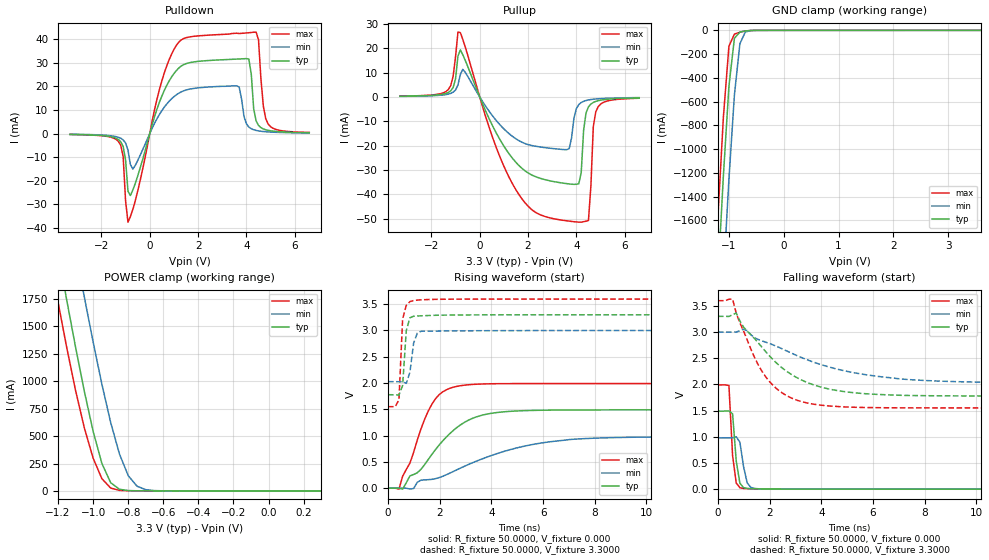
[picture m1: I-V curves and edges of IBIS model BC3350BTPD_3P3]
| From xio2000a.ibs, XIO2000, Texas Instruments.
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|   Model BC3350BTPD_3P3
[Model]   BC3350BTPD_3P3
Model_type   I/O
Polarity   Non-Inverting
Enable   Active-Low
Vinl =   0.9900V
Vinh =   2.3100V
Vmeas =   1.6500V
Cref =  15.0000pF
Rref = 100.0000M
Vref =  0.000V
C_comp   1.9708pF   2.0638pF   1.9731pF
[Model Spec]
|   typ   min   max
Vinh   2.31V   2.10V   2.52V
Vinl   0.99V   0.90V   1.08V
Vmeas   1.65V   1.50V   1.80V
[Temperature Range]   25.0000   0.1250k   -40.0000
[Voltage Range]   3.3000V   3.0000V   3.6000V
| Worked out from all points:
|   slope of the pulldown table from 0 to 0.495 V, typ, clamps not added: 31.4 ohm
|   slope of the pullup table from 0 to 0.495 V, typ, clamps not added: 44.5 ohm
|   GND clamp passes 1 mA (typ) near -0.59 V on its own axis
|   POWER clamp passes 1 mA (typ) near -0.74 V on its own axis
|   rising waveform, R_fixture 50.0000, V_fixture 0.000: 20-80 % time 1.63ns typ, 3.19ns min, 936ps max; typ from 0 V to 1.49 V
|   rising waveform, R_fixture 50.0000, V_fixture 3.3000: 20-80 % time 123ps typ, 174ps min, 113ps max; typ from 1.78 V to 3.3 V
|   falling waveform, R_fixture 50.0000, V_fixture 0.000: 20-80 % time 182ps typ, 214ps min, 166ps max; typ from 1.49 V to 0 V
|   falling waveform, R_fixture 50.0000, V_fixture 3.3000: 20-80 % time 2.06ns typ, 3.41ns min, 1.34ns max; typ from 3.3 V to 1.78 V
[Pulldown]
| voltage   I(typ)   I(min)   I(max)
-3.3V     -363uA     -290uA     -391uA
-1.3V     -2.499mA   -1.558mA   -3.272mA
-1.1V     -5.495mA   -2.672mA   -9.754mA
-900mV    -24.57mA   -7.086mA   -37.63mA
-700mV    -23.98mA   -15.08mA   -32.22mA
400mV     13.29mA    8.099mA    18.71mA
1.1V      26.74mA    16.46mA    37.45mA
3.6V      31.62mA    20.28mA    42.61mA
4.1V      31.65mA    2.775mA    42.82mA
4.4V      5.419mA    1.337mA    43.09mA
4.9V      1.364mA    701uA      4.046mA
6.6V      366uA      264uA      482uA
[Pullup]
| voltage   I(typ)   I(min)   I(max)
-3.3V     276uA      223uA      319uA
-1.3V     1.831mA    1.157mA    3.006mA
-800mV    19.29mA    9.256mA    26.38mA
600mV     -13.2mA    -8.655mA   -18.5mA
1.6V      -27.94mA   -17.82mA   -39.75mA
3.7V      -35.73mA   -21.26mA   -51mA
4.2V      -31.01mA   -2.304mA   -51.44mA
4.3V      -13.58mA   -1.804mA   -51.23mA
4.5V      -4.094mA   -1.249mA   -50.72mA
4.7V      -2.272mA   -950.1uA   -12.21mA
4.9V      -1.556mA   -765.1uA   -4.03mA
6.6V      -413uA     -285uA     -544uA
[GND_clamp]
| voltage   I(typ)   I(min)   I(max)
-3.3V     -22.46A    -23.25A    -22.02A
-1.3V     -2.981A    -3.864A    -2.466A
-1.2V     -2.075A    -2.956A    -1.561A
-1.1V     -1.216A    -2.078A    -723.4mA
-1V       -470.1mA   -1.253A    -133.5mA
-900mV    -66.75mA   -544.3mA   -31.76mA
-800mV    -14.28mA   -112.3mA   -15.85mA
-700mV    -5.191mA   -13.11mA   -5.235mA
-600mV    -1.114mA   -2.329mA   -804.1uA
-400mV    -42.11uA   -65.68uA   -59.17uA
3.6V      0A         0A         0A
[POWER_clamp]
| voltage   I(typ)   I(min)   I(max)
-3.3V     22.56A     23.38A     22.11A
-1.25V    2.627A     3.53A      2.158A
-1.2V     2.177A     3.077A     1.722A
-1.15V    1.736A     2.631A     1.304A
-1.05V    907.7mA    1.767A     573.9mA
-1V       543.7mA    1.358A     298.8mA
-950mV    250.4mA    972.4mA    111.3mA
-900mV    75.01mA    624.5mA    26.23mA
-850mV    15.11mA    336.8mA    5.041mA
-800mV    3.129mA    139.7mA    1.712mA
-750mV    1.084mA    43.46mA    1.075mA
300mV     0A         0A         0A
[Ramp]
| variable   typ   min   max
dV/dt_r   0.8935/1.6105n   0.5876/3.1587n   1.1937/0.9264n
dV/dt_f   0.9123/2.0434n   0.5823/3.3754n   1.2278/1.3245n
R_load = 50.0000
[Rising Waveform]
R_fixture = 50.0000
V_fixture = 0.000
V_fixture_min = 0.000
V_fixture_max = 0.000
| time   V(typ)   V(min)   V(max)
0s        1.533nV    33.95nV    723.3pV
424.2ps   2.21mV     -92.99uV   -18.02mV
565.7ps   -18.48mV   718.1uV    226.7mV
848.5ps   234.3mV    -16.16mV   476.1mV
1.273ns   357.1mV    151.2mV    1.122V
1.697ns   642.6mV    168mV      1.597V
2.546ns   1.106V     322.6mV    1.923V
3.818ns   1.408V     589.6mV    1.984V
6.364ns   1.485V     888.4mV    1.99V
14ns      1.489V     979.4mV    1.99V
[Rising Waveform]
R_fixture = 50.0000
V_fixture = 3.3000
V_fixture_min = 3.0000
V_fixture_max = 3.6000
| time   V(typ)   V(min)   V(max)
0s        1.777V     2.026V     1.55V
282.8ps   1.776V     2.026V     1.55V
424.2ps   1.77V      2.024V     1.684V
565.7ps   1.952V     2.026V     3.216V
707.1ps   2.997V     1.994V     3.477V
848.5ps   3.241V     2.205V     3.548V
989.9ps   3.27V      2.755V     3.568V
1.131ns   3.275V     2.946V     3.577V
1.273ns   3.278V     2.983V     3.582V
14ns      3.298V     2.999V     3.597V
[Falling Waveform]
R_fixture = 50.0000
V_fixture = 0.000
V_fixture_min = 0.000
V_fixture_max = 0.000
| time   V(typ)   V(min)   V(max)
0s        1.489V     980mV      1.99V
424.2ps   1.492V     980.8mV    1.979V
565.7ps   1.438V     980.6mV    642.4mV
707.1ps   536.2mV    999.8mV    117mV
848.5ps   113.7mV    896.6mV    26.96mV
989.9ps   28.44mV    431.7mV    13.77mV
1.131ns   13.59mV    119.6mV    9.799mV
1.273ns   9.73mV     34.67mV    6.845mV
1.414ns   7.8mV      13.6mV     4.945mV
14ns      495.4nV    5.95uV     264.7nV
[Falling Waveform]
R_fixture = 50.0000
V_fixture = 3.3000
V_fixture_min = 3.0000
V_fixture_max = 3.6000
| time   V(typ)   V(min)   V(max)
0s        3.298V     2.999V     3.597V
565.7ps   3.329V     2.998V     3.627V
707.1ps   3.361V     2.998V     3.357V
1.273ns   2.946V     2.947V     2.674V
1.838ns   2.628V     2.807V     2.15V
2.404ns   2.346V     2.696V     1.864V
3.253ns   2.078V     2.508V     1.668V
4.667ns   1.877V     2.284V     1.576V
7.071ns   1.791V     2.102V     1.552V
14ns      1.777V     2.028V     1.55V
